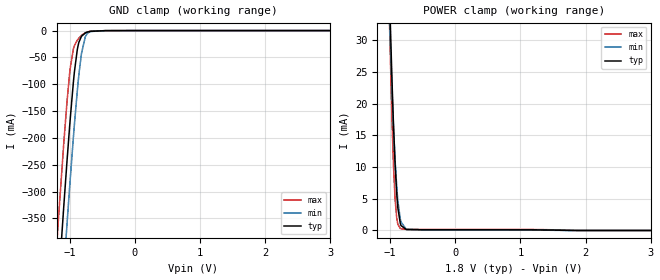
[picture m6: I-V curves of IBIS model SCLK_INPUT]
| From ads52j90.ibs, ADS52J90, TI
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|   Model
[Model]   SCLK_INPUT
Model_type   Input
Vinl = 0.45
Vinh = 1.35
|   typ   min   max
C_comp   1.431pF   1.417pF   1.444pF
[Voltage Range]   1.8   1.7   1.9
[Temperature Range]   25   85   -40
[Power Clamp Reference]   1.8   1.7   1.9
[GND Clamp Reference]   -0   -0   -0
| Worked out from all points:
|   GND clamp passes 1 mA (typ) near -0.61 V on its own axis
|   POWER clamp passes 1 mA (typ) near -0.84 V on its own axis
[GND Clamp]
|   Voltage   I(typ)   I(min)   I(max)
-1.8V     -1.671A    -1.791A    -1.551A
-1.195V   -518.1mA   -640mA     -395.6mA
-1.174V   -478.7mA   -600.5mA   -356.7mA
-1.087V   -325.1mA   -444.8mA   -207.5mA
-1.039V   -242.6mA   -359.8mA   -132mA
-990mV    -165.1mA   -277.6mA   -70.43mA
-941.4mV  -96.54mA   -199.5mA   -34.51mA
-882mV    -36.34mA   -113.7mA   -18.09mA
-817.2mV  -10.69mA   -42.95mA   -9.036mA
-757.8mV  -4.429mA   -11.34mA   -4.035mA
-450mV    -118.2uA   -91.2uA    -160.2uA
3.595V    0A         0A         0A
[POWER Clamp]
|   Voltage   I(typ)   I(min)   I(max)
-1.8V     409.6mA    346.2mA    478.3mA
-1.012V   37.67mA    33.69mA    33.38mA
-1.006V   35.65mA    32.03mA    31.02mA
-973.8mV  24.27mA    22.67mA    18.14mA
-957.6mV  19.17mA    18.46mA    12.76mA
-946.8mV  16.05mA    15.86mA    9.701mA
-925.2mV  10.62mA    11.24mA    5.025mA
-898.2mV  5.59mA     6.689mA    1.85mA
-882mV    3.55mA     4.663mA    988.1uA
-844.2mV  1.085mA    1.776mA    312.5uA
-752.4mV  146.6uA    179.5uA    175.5uA
3.595V    0A         0A         0A
